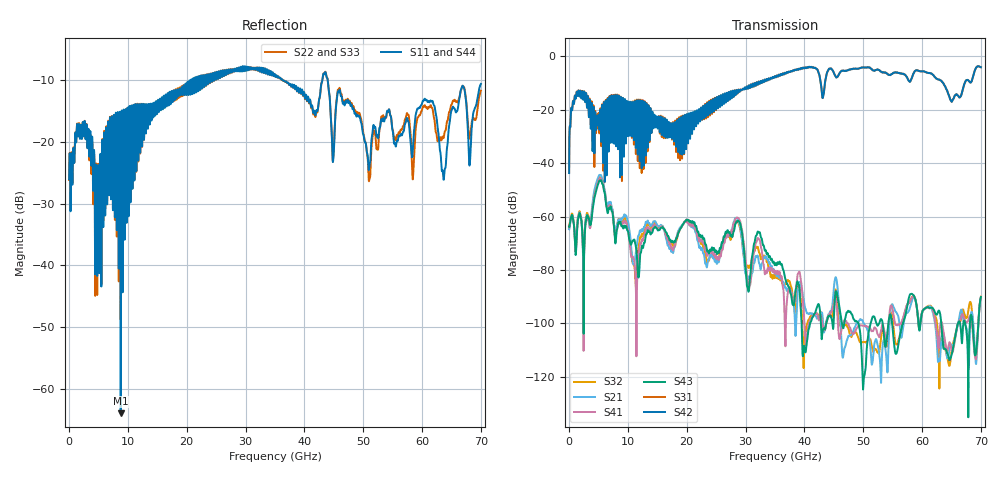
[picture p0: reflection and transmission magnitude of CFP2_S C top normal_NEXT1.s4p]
! AWR Design Environment (8415) Tue Jan 08 13:12:25 2019
! Document = 'CFP2 Channel_S'
! nPorts: 4, nXvals: 7001
# HZ S DB R 50
!Freq DBS11 AngS11 DBS12 AngS12 DBS13 AngS13 DBS14 AngS14
!	DBS21 AngS21 DBS22 AngS22 DBS23 AngS23 DBS24 AngS24
!	DBS31 AngS31 DBS32 AngS32 DBS33 AngS33 DBS34 AngS34
!	DBS41 AngS41 DBS42 AngS42 DBS43 AngS43 DBS44 AngS44
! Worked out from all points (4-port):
!   7000 points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, 10 MHz to 70 GHz, reference 50 ohm
!   strongest paths, dB at 10 MHz, 17.51 GHz, 35.01 GHz, 52.51 GHz, 70 GHz:
!     S42: -43.7, -30.5, -7.4, -5.0, -4.0
!     S31: -43.5, -31.2, -7.4, -5.0, -4.0
!     S43: -63.8, -69.1, -78.0, -100.7, -90.1
!     S41: -64.1, -71.6, -81.1, -104.2, -90.6
!     S21: -64.7, -72.5, -81.3, -108.4, -90.5
!     S32: -63.4, -69.9, -82.4, -110.8, -90.0
!   lowest |S11| = -63.9 dB at 8.78 GHz (marker M1), VSWR 1.00, Z = 50 + j0.058 ohm
!   |S11| at or under -10 dB: start of sweep to 20.78 GHz; 36.27 GHz to 43.07 GHz (6.797 GHz wide, 17.1 % of centre); 43.96 GHz to end of sweep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
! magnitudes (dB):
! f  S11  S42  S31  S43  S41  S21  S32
! 10 MHz  -26.1  -43.7  -43.5  -63.8  -64.1  -64.7  -63.4
! 1.34 GHz  -17.4  -13.3  -13.2  -66.0  -65.8  -64.3  -64.8
! 5.23 GHz  -26.0  -23.0  -22.3  -46.6  -45.8  -44.5  -45.1
! 8.78 GHz  -63.9  -15.9  -15.7  -62.4  -62.3  -61.1  -61.5
! 11.23 GHz  -14.4  -17.5  -17.2  -70.0  -80.1  -75.7  -81.6
! 28.55 GHz  -8.1  -13.3  -13.3  -61.6  -60.3  -60.6  -61.6
! 70 GHz  -10.7  -4.0  -4.0  -90.1  -90.6  -90.5  -90.0
